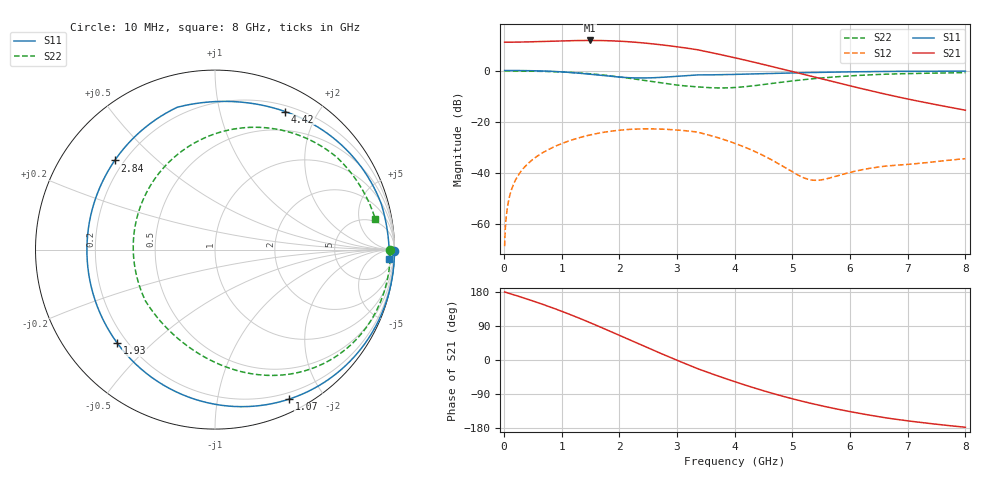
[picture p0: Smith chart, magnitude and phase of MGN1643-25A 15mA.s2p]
! Port[1] = GATE
! Port[2] = DRAIN
! [Type]  S-parameter s2p file touchstone ver. 1.0
! [Object]  MGN1643-25A
! [Bias]  15 mA
! [Version]  1.0
! [Date]  Tue May 19 13:03:48 2026
! [Source]  This file was created in JSC "ICC Milandr".
! [Disclaimer] Property of JSC "ICC Milandr". Unauthorized reproduction and/or distribution is strictly prohibited.
!  The file and the data are provided "AS IS" and with all faults and disclaim all warranties, express and implied, including
!  without limitation any implied warranties of merchantability, fitness for a particular purpose.
!  JSC "ICC Milandr" assumes no liability for:
!  1) the accuracy of the data provided;
!  2) the proper functioning of this data;
!  3) infringement of patents, copyrights or intellectual property rights resulting from the use of this data.
!  JSC "ICC Milandr" reserves the right to make changes to the products and the data without prior notice.
!  Please, be aware that your receipt and use of the file provided shall serve as acceptance of these terms and conditions.
!  If you do not accept these terms, you should return or destroy this file and any other accompanying information immediately.
# Hz S MA R 12.5
! freq  S11mag  S11ang  S21mag  S21ang  S12mag  S12ang  S22mag  S22ang
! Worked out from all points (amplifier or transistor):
!   800 points, 10 MHz to 8 GHz, reference 12.5 ohm
!   highest |S21| = 11.8 dB at 1.49 GHz (marker M1)
!   |S21| within 3 dB of that: start of sweep to 3.167 GHz
!   unconditionally stable (mu >= 1): 3.551 GHz to end of sweep
!   at 1.34 GHz: K = 0.36, MSG = 18.9 dB, |S12| = -26.1 dB
!   at 4.01 GHz: K = 1.61, MAG = 12.2 dB, |S12| = -28.6 dB
!   at 8 GHz: K = 1.51, MAG = 5.3 dB, |S12| = -34.6 dB
!   S11 on the Smith chart (normalised r, x): 10 MHz: open; 1.07 GHz: 0.13, -1.60; 1.93 GHz: 0.16, -0.39; 2.84 GHz: 0.16, +0.37; 4.42 GHz: 0.27, +1.60; 8 GHz: 15, -29
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1e7  0.9999 -0.5  3.588 179.5  0.0003606 83.4  0.9773 -0.3
1e8  1 -5.4  3.589 175.3  0.003576 85.1  0.9772 -3.0
2.6e8  0.9984 -14.1  3.608 167.7  0.009331 78.6  0.9758 -7.8
6.8e8  0.9781 -38.3  3.708 146.4  0.02485 59.2  0.9617 -20.8
1.07e9  0.9295 -63.7  3.822 124.5  0.03961 39.1  0.9284 -33.8
1.35e9  0.8762 -84.6  3.875 107.5  0.0498 23.4  0.889 -43.8
1.49e9  0.8455 -96.1  3.883 98.7  0.05451 15.2  0.8641 -49.0
1.71e9  0.7966 -115.4  3.86 84.4  0.06107 1.8  0.8185 -57.4
1.93e9  0.7536 -136.3  3.79 69.7  0.06625 -11.8  0.7665 -66.1
2.32e9  0.7144 -175.0  3.55 43.6  0.07134 -36.4  0.6674 -82.7
2.5e9  0.7164 167.7  3.401 31.7  0.07187 -47.6  0.6227 -91.1
2.68e9  0.7293 151.5  3.235 19.9  0.07135 -58.8  0.5809 -100.3
2.84e9  0.7475 138.4  3.079 9.6  0.07011 -68.6  0.5476 -109.2
3.09e9  0.7828 120.2  2.827 -6.3  0.06692 -83.8  0.5058 -125.1
3.38e9  0.8203 102.8  2.519 -24.2  0.06093 -100.8  0.4769 -146.5
3.68e9  0.8254 88.9  2.138 -40.6  0.04931 -113.9  0.4563 -170.1
4.01e9  0.8396 76.2  1.77 -57.7  0.03711 -126.2  0.4651 162.3
4.42e9  0.863 63.0  1.38 -77.5  0.02374 -136.9  0.5174 130.5
4.85e9  0.8884 51.3  1.049 -96.3  0.01299 -136.9  0.5969 103.2
5.34e9  0.914 39.9  0.763 -115.1  0.007129 -103.3  0.6872 79.3
6.67e9  0.9607 15.4  0.3327 -153.8  0.01357 -62.9  0.8525 36.9
8e9  0.9722 -3.1  0.1667 -177.5  0.01871 -85.6  0.9093 10.8
